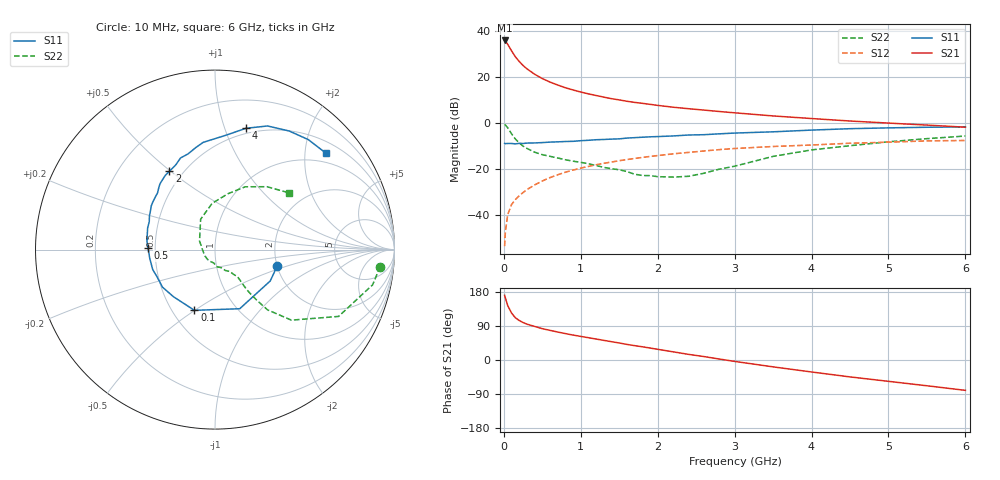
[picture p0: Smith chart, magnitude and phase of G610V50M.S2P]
! SIEMENS Small Signal Semiconductors
! BFG193
! Si NPN RF Bipolar Junction Transistor in SOT223
! VCE = 10 V  IC = 50 mA
! Common Emitter S-Parameters:  August  1996
# GHz  S  MA  R  50
!  f  S11  S21  S12  S22
! GHz  MAG  ANG  MAG  ANG  MAG  ANG  MAG  ANG
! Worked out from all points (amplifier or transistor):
!   36 points, 10 MHz to 6 GHz, reference 50 ohm
!   highest |S21| = 35.8 dB at 10 MHz (marker M1)
!   |S21| within 3 dB of that: start of sweep to 73.72 MHz
!   unconditionally stable (mu >= 1): 489.9 MHz to 2.404 GHz
!   at 250 MHz: K = 0.89, MSG = 27.6 dB, |S12| = -30.3 dB
!   at 1.4 GHz: K = 1.04, MAG = 12.5 dB, |S12| = -17.0 dB
!   at 6 GHz: K = 0.89, MSG = 2.9 dB, |S12| = -7.7 dB
!   S11 on the Smith chart (normalised r, x): 10 MHz: 2.01, -0.41; 100 MHz: 0.64, -0.50; 500 MHz: 0.46, +0.01; 2 GHz: 0.42, +0.49; 4 GHz: 0.45, +1.18; 6 GHz: 0.75, +2.46
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0.01  0.359 -14.3  61.72 170.8  0.0021 85.4  0.9253 -5.9
0.02  0.3539 -29.6  59.91 163.8  0.0043 81.4  0.8997 -12.6
0.05  0.3571 -67.3  51 143.7  0.0101 72.1  0.7827 -28.4
0.1  0.3572 -108.7  36.81 124.0  0.0168 66.3  0.5796 -42.7
0.15  0.35 -131.4  27.27 111.4  0.0216 64.2  0.4457 -48.9
0.2  0.3597 -144.4  21.59 104.3  0.0261 65.9  0.3685 -50.4
0.25  0.3568 -155.0  17.65 98.8  0.0307 66.9  0.3119 -51.3
0.3  0.3644 -162.2  14.95 94.6  0.0355 67.3  0.2791 -51.6
0.4  0.3669 -172.5  11.41 88.6  0.0449 68.2  0.2311 -50.9
0.5  0.3733 178.5  9.166 82.7  0.0547 67.4  0.2041 -50.4
0.6  0.3823 172.7  7.708 78.2  0.0648 66.5  0.1876 -51.2
0.8  0.3942 162.2  5.802 69.7  0.0847 63.6  0.1583 -54.5
1.1  0.419 149.2  4.267 58.8  0.1133 58.8  0.1297 -63.7
1.6  0.4677 131.9  2.95 41.1  0.1598 48.1  0.0876 -88.4
2  0.5045 120.2  2.4 28.2  0.195 39.3  0.0679 -129.5
2.2  0.52 114.9  2.19 21.6  0.2126 34.7  0.0665 -148.0
2.8  0.5783 100.7  1.768 2.6  0.2624 21.0  0.0988 150.9
3.5  0.6398 84.6  1.416 -18.1  0.3071 3.9  0.1873 115.3
4  0.6974 75.7  1.243 -31.6  0.3308 -5.8  0.2588 93.4
4.5  0.7483 67.0  1.098 -44.6  0.3614 -15.9  0.3193 77.0
5.5  0.8036 49.7  0.896 -68.0  0.4069 -39.1  0.4547 50.4
6  0.8184 41.2  0.806 -80.1  0.4143 -52.4  0.5181 37.7
